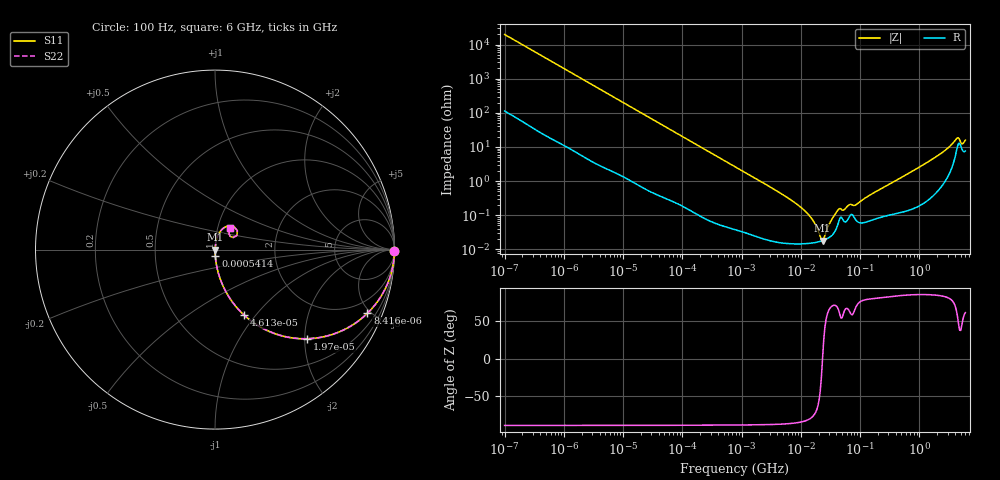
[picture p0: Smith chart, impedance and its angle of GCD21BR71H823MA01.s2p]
!Murata Part Number: GCD21BR71H823MA01
!These Parameters are Measured in Series Mode Connection
!Data Generated on Jan 08, 2026
!  o--ll--o
!Port1  Port2
!  o------o
!Operation Temp=25[degC], DC Bias Voltage=0[V]
!Freq. Start=100[Hz] Stop=6[GHz] 401[Steps]
# Hz S RI R 50
!Freq.(Hz) S11(Real) S11(Imag) S21(Real) S21(Imag) S12(Real) S12(Imag) S22(Real) S22(Imag)
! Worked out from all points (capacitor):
!   401 points, 100 Hz to 6 GHz, reference 50 ohm
!   read as one part in series: C = 80.2 nF near 109 Hz
!   lowest |Z| = 18 mohm at 23.28 MHz (marker M1)
!   series resonance near 23.25 MHz, so ESL is about 580 pH
!   S11 on the Smith chart (normalised r, x): 100 Hz: open; 8.416 kHz: 1.03, -4.78; 19.7 kHz: 1.01, -2.05; 46.13 kHz: 1.01, -0.88; 541.4 kHz: 1.00, -0.08; 6 GHz: 1.15, +0.28
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100  0.9999 -0.00505  5.45e-05 0.00505  5.45e-05 0.00505  0.9999 -0.00505
2008  0.9895 -0.0992  0.0105 0.0992  0.0105 0.0992  0.9895 -0.0992
8416  0.8494 -0.3544  0.1506 0.3544  0.1506 0.3544  0.8494 -0.3544
19704  0.512 -0.4965  0.488 0.4965  0.488 0.4965  0.512 -0.4965
40335  0.203 -0.3985  0.797 0.3985  0.797 0.3985  0.203 -0.3985
46134  0.1635 -0.366  0.8365 0.366  0.8365 0.366  0.1635 -0.366
141303  0.0216 -0.141  0.9784 0.141  0.9784 0.141  0.0216 -0.141
541393  0.00188 -0.0378  0.9981 0.0378  0.9981 0.0378  0.00188 -0.0378
774597  0.00108 -0.0265  0.9989 0.0265  0.9989 0.0265  0.00108 -0.0265
6948629  0.000153 -0.00273  0.9998 0.00273  0.9998 0.00273  0.000153 -0.00273
1.137099e7  0.000148 -0.0014  0.9999 0.0014  0.9999 0.0014  0.000148 -0.0014
1.555665e7  0.000154 -0.000748  0.9998 0.000748  0.9998 0.000748  0.000154 -0.000748
2.128304e7  0.000171 -0.000162  0.9998 0.000162  0.9998 0.000162  0.000171 -0.000162
2.327686e7  0.000179 1.8e-06  0.9998 -1.8e-06  0.9998 -1.8e-06  0.000179 1.8e-06
3.330331e7  0.000257 0.000709  0.9997 -0.000709  0.9997 -0.000709  0.000257 0.000709
4.35672e7  0.00064 0.00135  0.9994 -0.00135  0.9994 -0.00135  0.00064 0.00135
8.527865e7  0.000722 0.00188  0.9993 -0.00188  0.9993 -0.00188  0.000722 0.00188
3.124326e8  0.00107 0.00805  0.9989 -0.00805  0.9989 -0.00805  0.00107 0.00805
1.873145e9  0.00676 0.0495  0.9932 -0.0495  0.9932 -0.0495  0.00676 0.0495
4.193612e9  0.0845 0.1329  0.9155 -0.1329  0.9155 -0.1329  0.0845 0.1329
5.245841e9  0.0853 0.0735  0.9147 -0.0735  0.9147 -0.0735  0.0853 0.0735
6e9  0.0862 0.1192  0.9138 -0.1192  0.9138 -0.1192  0.0862 0.1192
